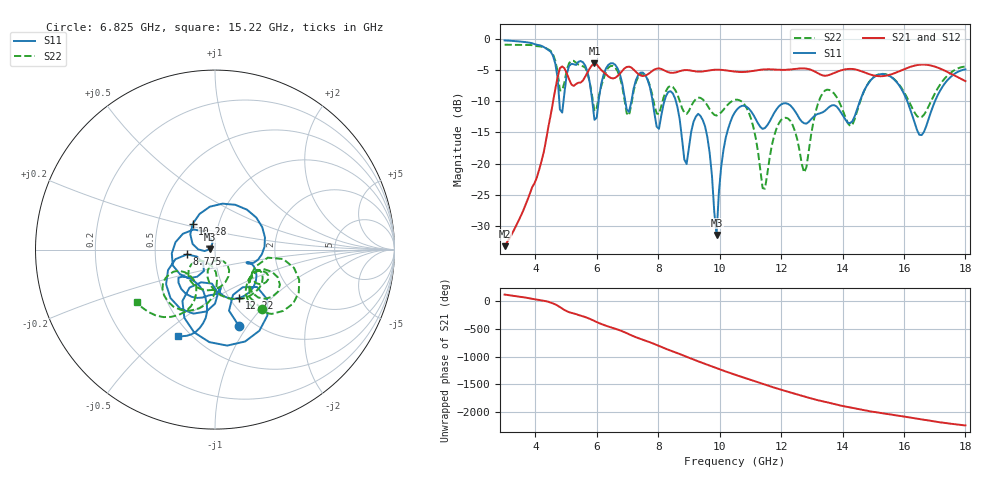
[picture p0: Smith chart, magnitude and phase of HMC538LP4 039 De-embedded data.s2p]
! Chelmsford, MA 01824
! http://www.hittite.com
! Tel: 978-250-3343
! Fax: 978-250-3373
! Device  :  HMC538LP4
! Description:  600 Analog Phase Shifter
! Frequency  :  6.0 GHz - 15.0 GHz
! Package  :  LP4  - 4x4 mm Quad Flatpack No-Lead (QFN) Plastic Package: 24 pin
! Ports  :  2 RF, 1 DC
!  Pin  3  = Rfin  = Port 1
!  Pin  16  = Rfout = Port 2
!  pin  21  = vCTL
! Voltages:  VCTL  = 0 to 5.0 Volts
! Currents :  Vb(V)  Vd(V)  Ib(mA)  Id(mA)
!  0.00  3.90  0.000000	0.474412
! Data:  The device was measured on evaluation board 111296-1.
!  Data was collected using a calibrated network analyzer.
!  The evaluation circuit board was modeled and simulated.This was use
!  to removed the evaluation board circuit from the measured data.
!  The reference plane is the center of the package pin.
! Misc:  Lot #
!Date Measured:  03 - 11 -2009
! Date:  03 - 17 -2009
! Note:
!  Hittite Microwave supplies this data as a sample of measured data at the
!  package pin for this package product.  Your particular data for this product
!  may vary.
!  Data was taken at 25 degrees C.
!  Hittite Microwave reserves the right to change this data at anytime.
# MHz S MA R 50
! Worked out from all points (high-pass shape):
!   201 points, 3 GHz to 18 GHz, reference 50 ohm
!   highest |S21| = -3.90 dB at 5.925 GHz (marker M1); lowest = -33.3 dB at 3 GHz (marker M2)
!   |S21| within 3 dB of the highest: 4.694 GHz to 5.141 GHz (446.8 MHz wide, 9.09 % of centre); 5.491 GHz to end of sweep
!   lowest |S11| = -31.5 dB at 9.9 GHz (marker M3), VSWR 1.05, Z = 47.4 + j0.282 ohm
!   |S11| at or under -10 dB: 7.818 GHz to 8.2 GHz (381.9 MHz wide, 4.77 % of centre); 8.576 GHz to 14.56 GHz (5.988 GHz wide, 51.8 % of centre); 16.11 GHz to 17.01 GHz (898.9 MHz wide, 5.43 % of centre)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
!   |S22| runs from -24.1 to -0.9 dB; largest |S21 - S12| = 0.0028
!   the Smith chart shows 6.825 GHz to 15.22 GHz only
!   S11 on the Smith chart (normalised r, x): 6.825 GHz: 0.86, -0.92; 8.775 GHz: 0.73, -0.04; 10.28 GHz: 0.75, +0.22; 12.22 GHz: 1.11, -0.66; 15.22 GHz: 0.43, -0.57
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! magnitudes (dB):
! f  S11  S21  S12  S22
! 3 GHz  -0.2  -33.3  -33.3  -0.9
! 4.5 GHz  -2.0  -12.2  -12.2  -1.9
! 4.8 GHz  -11.3  -4.7  -4.7  -8.2
! 5.55 GHz  -3.7  -6.6  -6.6  -4.3
! 5.925 GHz  -13.0  -3.9  -3.9  -11.6
! 6.825 GHz  -7.0  -5.1  -5.1  -7.5
! 7.575 GHz  -5.7  -5.9  -5.9  -5.8
! 8.025 GHz  -14.4  -4.7  -4.7  -12.1
! 8.4 GHz  -8.4  -5.4  -5.4  -7.5
! 8.775 GHz  -16.0  -5.0  -5.0  -11.1
! 9.525 GHz  -14.0  -5.1  -5.1  -10.1
! 9.9 GHz  -31.5  -4.9  -4.9  -12.3
! 10.28 GHz  -14.4  -5.1  -5.1  -10.5
! 10.5 GHz  -11.7  -5.2  -5.2  -9.7
! 11.4 GHz  -14.4  -4.9  -4.9  -24.0
! 12.22 GHz  -10.4  -4.9  -4.9  -12.7
! 12.75 GHz  -13.5  -4.7  -4.7  -21.4
! 13.05 GHz  -12.5  -5.1  -5.1  -13.4
! 15.22 GHz  -5.6  -6.0  -6.0  -5.6
! 15.53 GHz  -5.9  -5.7  -5.8  -5.9
! 16.57 GHz  -15.4  -4.1  -4.1  -12.5
! 18 GHz  -4.8  -6.7  -6.8  -4.4
